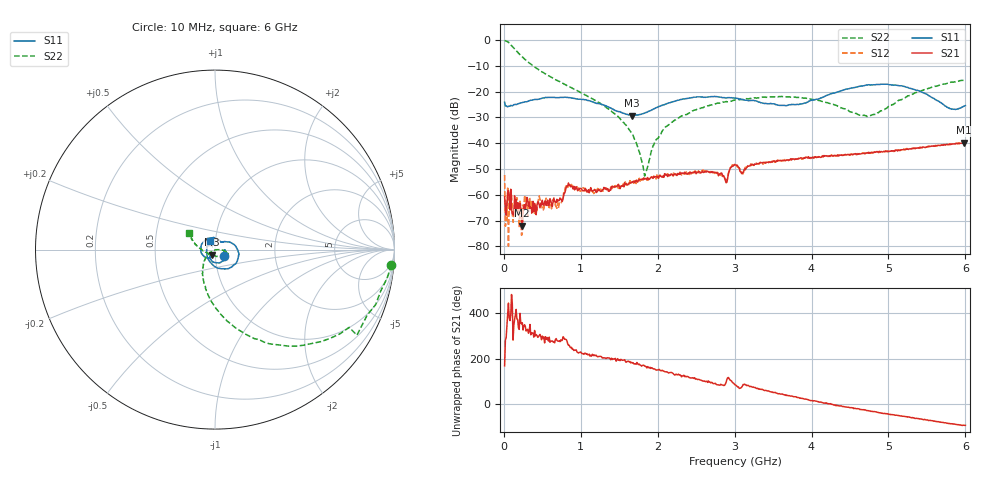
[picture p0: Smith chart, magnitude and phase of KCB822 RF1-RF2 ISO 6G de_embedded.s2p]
!Agilent	"Technologies,N5230A,MY45001650,A.07.50.48"
!Agilent	N5230A:	A.07.50.48
!Date:	"Tuesday,"	April	"29,"	2014	13:35:06
!Correction:	S11(Full	2	"Port(1,2))"
!S21(Full	2	"Port(1,2))"
!S12(Full	2	"Port(1,2))"
!S22(Full	2	"Port(1,2))"
!S2P	File:	Measurements:	"S11,"	"S21,"	"S12,"	S22:
#	Hz	S	dB	R	50
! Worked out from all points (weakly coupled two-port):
!   600 points, 10 MHz to 6 GHz, reference 50 ohm
!   highest |S21| = -39.80 dB at 5.98 GHz (marker M1); lowest = -72.0 dB at 240 MHz (marker M2)
!   lowest |S11| = -29.3 dB at 1.67 GHz (marker M3), VSWR 1.07, Z = 48.1 - j2.8 ohm
!   |S11| at or under -10 dB: start of sweep to end of sweep
!   |S22| runs from -52.7 to -0.1 dB; largest |S21 - S12| = 0.0033
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1e7  -24.10 -33.0  -60.70 168.0  -52.30 -1.9  -0.12 -5.0
5e7  -25.90 -8.6  -59.70 36.9  -57.40 86.2  -0.69 -23.2
8e7  -25.60 -3.4  -65.90 7.4  -64.50 -65.3  -1.52 -34.0
2.4e8  -24.20 -9.5  -72.00 -2.0  -74.90 51.8  -6.52 -73.0
4.7e8  -22.80 -32.2  -65.00 -53.5  -62.00 -43.8  -11.80 -98.4
7.1e8  -22.30 -60.2  -62.10 -83.1  -65.10 -78.5  -15.90 -115.0
8.4e8  -22.30 -73.9  -55.40 -101.0  -56.40 -97.9  -17.90 -122.0
1.01e9  -23.00 -94.6  -57.70 -136.0  -58.40 -144.0  -20.50 -131.0
1.46e9  -27.40 -128.0  -56.70 -171.0  -57.30 -164.0  -29.10 -148.0
1.67e9  -29.30 -122.0  -55.20 -179.0  -54.90 -175.0  -36.50 -149.0
1.84e9  -28.20 -115.0  -53.80 167.0  -53.20 162.0  -51.60 -62.4
2.01e9  -25.80 -120.0  -53.50 152.0  -53.60 154.0  -37.80 3.6
2.31e9  -23.00 -146.0  -51.70 120.0  -52.30 129.0  -29.40 -0.2
2.88e9  -22.40 143.0  -54.60 88.6  -54.10 85.0  -23.90 -13.2
3.01e9  -22.50 126.0  -48.40 84.4  -48.50 83.7  -23.20 -13.9
3.1e9  -23.10 116.0  -51.80 78.5  -51.60 83.3  -23.00 -17.0
4.01e9  -23.30 41.4  -45.60 15.7  -45.20 15.8  -23.00 -35.7
4.72e9  -17.40 -9.5  -43.70 -28.8  -43.60 -29.9  -29.60 -108.0
5.01e9  -17.30 -36.8  -43.20 -45.6  -43.20 -45.1  -25.50 -163.0
5.81e9  -26.60 -172.0  -40.40 -86.7  -40.40 -85.4  -16.30 153.0
5.98e9  -25.60 128.0  -39.80 -93.2  -39.90 -93.4  -15.60 148.0
6e9  -25.40 122.0  -39.80 -93.6  -39.80 -94.6  -15.40 147.0
